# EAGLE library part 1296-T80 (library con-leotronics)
1.27mm SINGLE ROW FEMALE SOCKET Source: http://www.leotronics.co.uk/Conexcon/Data%20Sheets/sec.%20A/1296ing.pdf
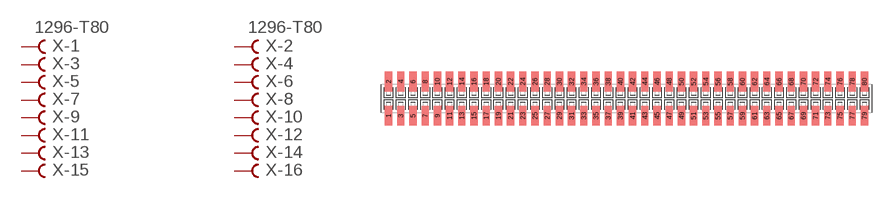
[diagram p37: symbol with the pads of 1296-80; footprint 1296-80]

Designator prefix X; gates -1=FVAL -2=FVAL -3=F -4=F -5=F -6=F -7=F -8=F -9=F -10=F -11=F -12=F -13=F -14=F -15=F -16=F -17=F -18=F -19=F -20=F -21=F -22=F -23=F -24=F -25=F -26=F -27=F -28=F -29=F -30=F -31=F -32=F -33=F -34=F -35=F -36=F -37=F -38=F -39=F -40=F -41=F -42=F -43=F -44=F -45=F -46=F -47=F -48=F -49=F -50=F -51=F -52=F -53=F -54=F -55=F -56=F -57=F -58=F -59=F -60=F -61=F -62=F -63=F -64=F -65=F -66=F -67=F -68=F -69=F -70=F -71=F -72=F -73=F -74=F -75=F -76=F -77=F -78=F -79=F -80=F

## 1296-T80 (OC_FARNELL: unknown; OC_NEWARK: unknown)  [1296-80]
1  -1:B  pas
2  -2:B  pas
3  -3:B  pas
4  -4:B  pas
5  -5:B  pas
6  -6:B  pas
7  -7:B  pas
8  -8:B  pas
9  -9:B  pas
10  -10:B  pas
11  -11:B  pas
12  -12:B  pas
13  -13:B  pas
14  -14:B  pas
15  -15:B  pas
16  -16:B  pas
17  -17:B  pas
18  -18:B  pas
19  -19:B  pas
20  -20:B  pas
21  -21:B  pas
22  -22:B  pas
23  -23:B  pas
24  -24:B  pas
25  -25:B  pas
26  -26:B  pas
27  -27:B  pas
28  -28:B  pas
29  -29:B  pas
30  -30:B  pas
31  -31:B  pas
32  -32:B  pas
33  -33:B  pas
34  -34:B  pas
35  -35:B  pas
36  -36:B  pas
37  -37:B  pas
38  -38:B  pas
39  -39:B  pas
40  -40:B  pas
41  -41:B  pas
42  -42:B  pas
43  -43:B  pas
44  -44:B  pas
45  -45:B  pas
46  -46:B  pas
47  -47:B  pas
48  -48:B  pas
49  -49:B  pas
50  -50:B  pas
51  -51:B  pas
52  -52:B  pas
53  -53:B  pas
54  -54:B  pas
55  -55:B  pas
56  -56:B  pas
57  -57:B  pas
58  -58:B  pas
59  -59:B  pas
60  -60:B  pas
61  -61:B  pas
62  -62:B  pas
63  -63:B  pas
64  -64:B  pas
65  -65:B  pas
66  -66:B  pas
67  -67:B  pas
68  -68:B  pas
69  -69:B  pas
70  -70:B  pas
71  -71:B  pas
72  -72:B  pas
73  -73:B  pas
74  -74:B  pas
75  -75:B  pas
76  -76:B  pas
77  -77:B  pas
78  -78:B  pas
79  -79:B  pas
80  -80:B  pas

## Footprint 1296-80 (pad centres in mm)
1.27mm SINGLE ROW FEMALE SOCKET Source: http://www.leotronics.co.uk/Conexcon/Data%20Sheets/sec.%20A/1296ing.pdf
smd 0.76 x 2.05: 1 -24.765,-1.78; 2 -24.765,1.78; 3 -23.495,-1.78; 4 -23.495,1.78; 5 -22.225,-1.78; 6 -22.225,1.78; 7 -20.955,-1.78; 8 -20.955,1.78; 9 -19.685,-1.78; 10 -19.685,1.78; 11 -18.415,-1.78; 12 -18.415,1.78; 13 -17.145,-1.78; 14 -17.145,1.78; 15 -15.875,-1.78; 16 -15.875,1.78; 17 -14.605,-1.78; 18 -14.605,1.78; 19 -13.335,-1.78; 20 -13.335,1.78; 21 -12.065,-1.78; 22 -12.065,1.78; 23 -10.795,-1.78; 24 -10.795,1.78; 25 -9.525,-1.78; 26 -9.525,1.78; 27 -8.255,-1.78; 28 -8.255,1.78; 29 -6.985,-1.78; 30 -6.985,1.78; 31 -5.715,-1.78; 32 -5.715,1.78; 33 -4.445,-1.78; 34 -4.445,1.78; 35 -3.175,-1.78; 36 -3.175,1.78; 37 -1.905,-1.78; 38 -1.905,1.78; 39 -0.635,-1.78; 40 -0.635,1.78; 41 0.635,-1.78; 42 0.635,1.78; 43 1.905,-1.78; 44 1.905,1.78; 45 3.175,-1.78; 46 3.175,1.78; 47 4.445,-1.78; 48 4.445,1.78; 49 5.715,-1.78; 50 5.715,1.78; 51 6.985,-1.78; 52 6.985,1.78; 53 8.255,-1.78; 54 8.255,1.78; 55 9.525,-1.78; 56 9.525,1.78; 57 10.795,-1.78; 58 10.795,1.78; 59 12.065,-1.78; 60 12.065,1.78; 61 13.335,-1.78; 62 13.335,1.78; 63 14.605,-1.78; 64 14.605,1.78; 65 15.875,-1.78; 66 15.875,1.78; 67 17.145,-1.78; 68 17.145,1.78; 69 18.415,-1.78; 70 18.415,1.78; 71 19.685,-1.78; 72 19.685,1.78; 73 20.955,-1.78; 74 20.955,1.78; 75 22.225,-1.78; 76 22.225,1.78; 77 23.495,-1.78; 78 23.495,1.78; 79 24.765,-1.78; 80 24.765,1.78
